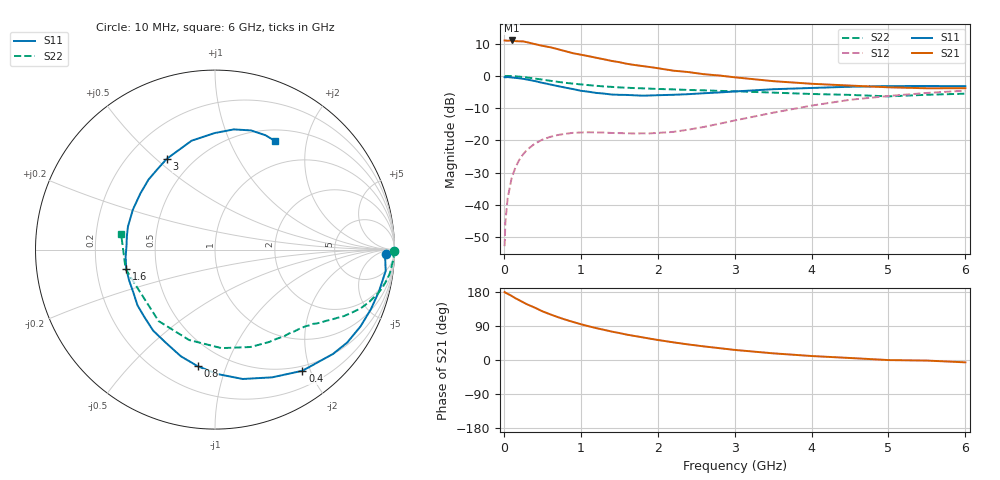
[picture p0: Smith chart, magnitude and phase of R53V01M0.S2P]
! SIEMENS Small Signal Semiconductors
! BFR183
! Si NPN RF Bipolar Junction Transistor in SOT23
! VCE = 3 V  IC = 1 mA
! Common Emitter S-Parameters:  May  1996
# GHz  S  MA  R  50
!  f  S11  S21  S12  S22
! GHz  MAG  ANG  MAG  ANG  MAG  ANG  MAG  ANG
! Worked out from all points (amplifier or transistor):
!   36 points, 10 MHz to 6 GHz, reference 50 ohm
!   highest |S21| = 11.0 dB at 100 MHz (marker M1)
!   |S21| within 3 dB of that: start of sweep to 749.3 MHz
!   unconditionally stable (mu >= 1): 1.656 GHz to 2.951 GHz
!   at 250 MHz: K = 0.15, MSG = 17.5 dB, |S12| = -24.3 dB
!   at 1.4 GHz: K = 0.86, MSG = 11.2 dB, |S12| = -17.7 dB
!   at 6 GHz: K = 0.95, MSG = 0.4 dB, |S12| = -4.6 dB
!   S11 on the Smith chart (normalised r, x): 10 MHz: 33, -17; 400 MHz: 0.43, -1.88; 800 MHz: 0.35, -0.80; 1.6 GHz: 0.33, -0.10; 3 GHz: 0.36, +0.54; 6 GHz: 0.65, +1.50
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0.01  0.9532 -1.4  3.533 179.3  0.0023 93.3  0.9994 -0.5
0.02  0.9492 -2.9  3.522 177.7  0.0054 90.3  0.9921 -1.0
0.05  0.9584 -7.1  3.501 174.7  0.0128 84.7  0.9971 -2.6
0.1  0.9428 -14.3  3.535 169.3  0.0256 82.0  0.9889 -5.1
0.15  0.9299 -20.9  3.455 163.1  0.038 77.2  0.9827 -7.8
0.25  0.9004 -35.1  3.42 152.4  0.0608 69.2  0.9582 -12.5
0.3  0.8775 -41.5  3.321 147.1  0.0713 65.6  0.9429 -14.7
0.4  0.8324 -54.2  3.109 138.4  0.0887 58.8  0.9097 -18.5
0.5  0.7797 -65.9  2.923 128.6  0.1027 52.7  0.8758 -21.9
0.6  0.7372 -77.9  2.779 120.7  0.1133 47.6  0.8397 -24.7
0.8  0.6571 -98.4  2.411 106.5  0.1268 39.5  0.78 -29.2
0.9  0.6238 -107.8  2.241 100.4  0.131 36.6  0.7582 -30.9
1.1  0.5681 -127.3  2.02 89.2  0.1337 32.3  0.7183 -34.3
1.4  0.5138 -152.3  1.704 75.1  0.1304 30.2  0.6749 -38.7
1.6  0.5062 -167.7  1.537 66.9  0.1289 31.5  0.6544 -41.4
1.9  0.4965 171.6  1.369 56.3  0.1285 36.9  0.6339 -46.1
2.2  0.5089 154.1  1.205 46.7  0.1355 44.2  0.6178 -51.3
3  0.5729 117.9  0.95 26.6  0.2036 56.9  0.5772 -70.1
3.5  0.6207 102.1  0.828 17.6  0.2687 55.8  0.5502 -86.2
4.5  0.6779 81.1  0.707 5.3  0.4258 42.6  0.5072 -128.3
5.5  0.6964 66.1  0.642 -1.5  0.5437 25.4  0.5096 -167.7
6  0.6914 60.9  0.644 -6.2  0.5899 15.3  0.5297 170.7
